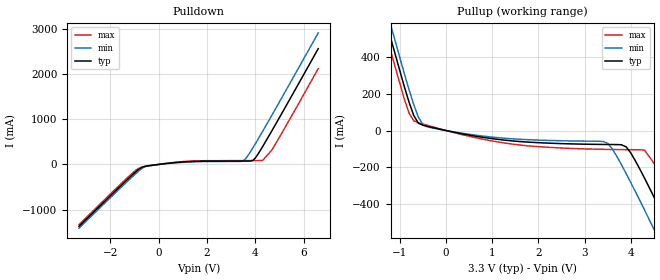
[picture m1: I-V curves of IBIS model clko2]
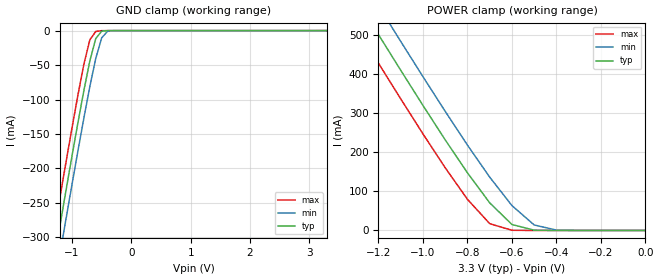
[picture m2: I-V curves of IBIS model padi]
|   * 91305s3.ibs * IBIS 1.1 Model for ICS91305
| Rev History
| Rev No.   Description
| 1.0   Initial release with Updated Parasitic Parameters
[IBIS Ver]	1.1
[Comment char]	|_char
[File name]	91305s3.ibs
[Date]		Fri 15:30 July 27, 2001
[File Rev]	1.0
[Source] 	Originated at Integrated Circuit Systems, Inc.
[Disclaimer]
(C) Copyright Integrated Circuit Systems, Inc. 1997
   All rights reserved
ICS hereby grants the user of this IBIS model a non-exclusive,
nontransferable license to use this IBIS model under the following terms.
Before using this IBIS model, the user should read this license.
If the user does not accept these terms,  the IBIS model should be
returned to ICS within 30 days.
   The user is granted this license only to use the IBIS model and
is not granted rights to sell, load, rent, lease or license the IBIS
model in whole or in part, or in modified form to anyone other than
user. User may modify the IBIS model to suit its specific
applications but rights to derivative works and such modifications
shall belong to ICS.
   This IBIS model is provided on an "AS IS" basis and ICS makes
absolutely no warranty with respect to the information contained
herein. ICS DISCLAIMS AND CUSTOMER WAIVES ALL WARRANTIES, EXPRESS
OR IMPLIED, INCLUDING WARRANTIES OF MERCHANTABILITY OR FITNESS FOR
A PARTICULAR PURPOSE. The entire risk as to quality and performance
is with the Customer. ACCORDINGLY, IN NO EVENT SHALL THE COMPANY BE
LIABLE FOR ANY DAMAGES, WHETHER IN CONTRACT OR TORT,INCLUDING ANY
LOST PROFITS OR OTHER INCIDENTAL, CONSEQUENTIAL, EXEMPLARY, OR
PUNITIVE DAMAGES ARISING OUT OF THE USE OR APPLICATION OF THE IBIS
model provided in this package. Further, ICS reserves the right to
make changes without notice to any product herein to improve
reliability, function, or design. ICS does not convey any license
under patent rights or any other intellectual property rights,
including those of third parties.
   ICS is not obligated to provide maintenance or support
for the licensed IBIS model.
|   COMPONENT: ICS91305
[Component]	ICS91305
[Manufacturer]	ICS
[Package]
| variable	typ	min	max
R_pkg   37.6m   32.9m   42.3m
L_pkg   3.1nH   2.6nH   3.6nH
C_pkg   0.34pF  0.14pF  0.54pF
[Pin]	signal_name		model_name	R_pin	L_pin	C_pin
1	REF			padi
2	CLK2			clko2
3	CLK1			clko2
4	GND			GND
5	CLK3			clko2
6	VDD			POWER
7	CLK4			clko2
8	CLKOUT		clko2
| Models and submodels in the file (2): clko2 (Output), padi (Input)
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|   MODEL clko2
[Model]		clko2
Model_type	Output
Polarity	Non-Inverting
C_comp   5.5pF   5.0pF   6.0pF
[Voltage range]   3.300   3.000   3.700
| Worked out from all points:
|   slope of the pulldown table from 0 to 0.495 V, typ, clamps not added: 16.2 ohm
|   slope of the pullup table from 0 to 0.495 V, typ, clamps not added: 20.2 ohm
[Pulldown]
|  Voltage   I(typ)   I(min)   I(max)
-3.3V     -1.37A     -1.41A     -1.331A
-1V       -187mA     -226.4mA   -150.2mA
-800mV    -98.35mA   -132.5mA   -80.99mA
-600mV    -45.96mA   -55.11mA   -50.13mA
1.1V      57.01mA    49.12mA    66.49mA
3.5V      74.31mA    79.9mA     83.99mA
3.8V      75.34mA    284.3mA    84.35mA
3.9V      89.95mA    370.7mA    84.46mA
4V        145.4mA    459.4mA    84.58mA
4.3V      394.6mA    732.8mA    87.51mA
4.7V      760.5mA    1.105A     332.4mA
6.6V      2.561A     2.909A     2.119A
[Pullup]
|  Voltage   I(typ)   I(min)   I(max)
-3.3V     2.484A     2.555A     2.415A
-1.3V     594.4mA    667.6mA    522.1mA
-800mV    154mA      222mA      94.72mA
-600mV    40.2mA     73.06mA    42.67mA
600mV     -29.06mA   -23.87mA   -36.82mA
3.5V      -76.19mA   -69.44mA   -103mA
3.9V      -88.59mA   -233.8mA   -104.4mA
4.3V      -259.6mA   -433.2mA   -106.6mA
4.7V      -461.1mA   -638.3mA   -247.2mA
5.1V      -667.3mA   -845.6mA   -448.7mA
5.5V      -875.5mA   -1.054A    -655.5mA
6.6V      -1.452A    -1.631A    -1.232A
[Ramp]
|  variable   typ   min   max
dV/dt_r   1.36/0.29n   1.14/0.33n   1.65/0.27n
dV/dt_f   1.46/0.28n   1.27/0.30n   1.70/0.28n
|   MODEL padi
[Model]		padi
Model_type	Input
C_comp   5.5pF   5.0pF   6.0pF
[Voltage range]   3.300   3.000   3.700
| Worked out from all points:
|   GND clamp passes 1 mA (typ) near -0.50 V on its own axis
|   POWER clamp passes 1 mA (typ) near -0.50 V on its own axis
[GND_clamp]
|  Voltage   I(typ)   I(min)   I(max)
-3.3V     -1.37A     -1.409A    -1.331A
-1.3V     -331.8mA   -373.2mA   -290.8mA
-1.2V     -281.3mA   -322.7mA   -240.2mA
-1.1V     -231.2mA   -272.6mA   -190.2mA
-900mV    -133.5mA   -174.4mA   -93.39mA
-800mV    -86.94mA   -126.8mA   -48.84mA
-700mV    -44.15mA   -81.44mA   -13.49mA
-600mV    -11.56mA   -40.46mA   -1.257mA
-500mV    -795uA     -10.56mA   -77.54uA
-400mV    -27.71uA   -852.7uA   -1.223uA
3.3V      227.9pA    44.02uA    159.3pA
[POWER_clamp]
|  Voltage   I(typ)   I(min)   I(max)
-3.3V     2.484A     2.554A     2.415A
-1.3V     592.5mA    666.2mA    519.5mA
-1.2V     500.5mA    574.3mA    427.4mA
-1.1V     409.4mA    483.1mA    336.3mA
-900mV    231.5mA    304.4mA    160.2mA
-800mV    147.3mA    218.1mA    79.55mA
-700mV    70.56mA    136.3mA    17.43mA
-600mV    15.25mA    63.53mA    531.6uA
-500mV    728.2uA    14mA       8.075uA
-400mV    20.89uA    955uA      118.3nA
0V        227.9pA    10.63nA    207.3pA
